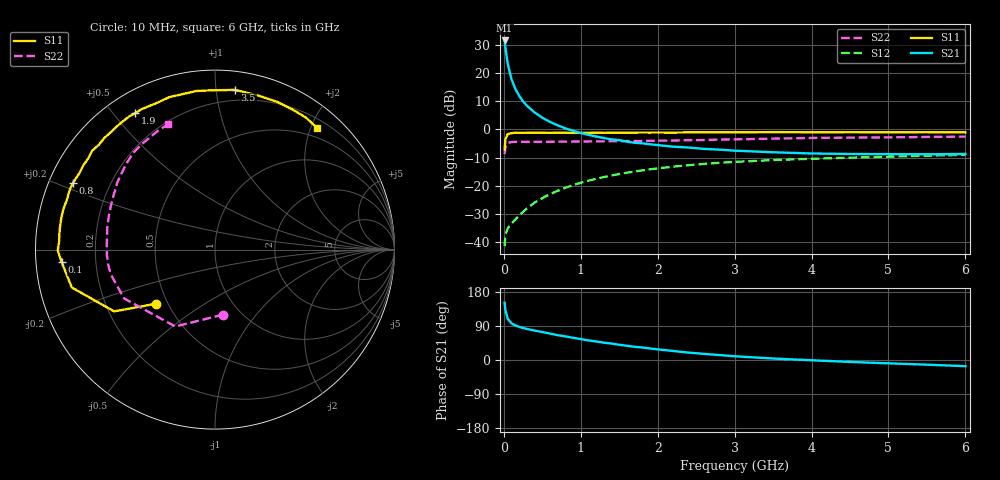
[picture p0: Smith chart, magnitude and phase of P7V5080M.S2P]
! SIEMENS Small Signal Semiconductors
! BFP196
! Si NPN RF Bipolar Junction Transistor in SOT143
! VCE = 0.5 V  IC = 80 mA
! Common Emitter S-Parameters:  May  1996
# GHz  S  MA  R  50
!  f  S11  S21  S12  S22
! GHz  MAG  ANG  MAG  ANG  MAG  ANG  MAG  ANG
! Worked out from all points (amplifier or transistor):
!   36 points, 10 MHz to 6 GHz, reference 50 ohm
!   highest |S21| = 31.7 dB at 10 MHz (marker M1)
!   |S21| within 3 dB of that: start of sweep to 23.11 MHz
!   unconditionally stable (mu >= 1): start of sweep to 13.67 MHz; 160.8 MHz to end of sweep
!   at 250 MHz: K = 1.19, MAG = 17.1 dB, |S12| = -29.4 dB
!   at 1.4 GHz: K = 1.27, MAG = 3.3 dB, |S12| = -16.4 dB
!   at 6 GHz: K = 1.09, MAG = -1.7 dB, |S12| = -9.1 dB
!   S11 on the Smith chart (normalised r, x): 10 MHz: 0.43, -0.33; 100 MHz: 0.08, -0.04; 800 MHz: 0.07, +0.22; 1.9 GHz: 0.08, +0.57; 3.5 GHz: 0.12, +1.12; 6 GHz: 0.33, +2.09
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0.01  0.4441 -137.3  38.64 151.0  0.0083 56.5  0.3649 -82.9
0.02  0.659 -148.5  29.32 131.8  0.0131 44.1  0.4823 -117.3
0.05  0.8254 -165.2  14.99 108.7  0.0173 35.7  0.575 -151.8
0.1  0.8572 -175.4  7.805 96.7  0.0211 41.6  0.5967 -166.6
0.15  0.8761 -179.6  5.272 91.2  0.0248 46.9  0.601 -171.9
0.2  0.8697 177.1  3.967 87.3  0.0293 52.7  0.6013 -174.9
0.25  0.8713 174.5  3.167 84.4  0.034 56.1  0.6032 -177.1
0.3  0.8727 172.5  2.649 82.1  0.039 58.8  0.6023 -178.5
0.4  0.8743 168.2  2.006 77.6  0.0497 61.6  0.6032 179.2
0.5  0.8744 165.1  1.622 73.8  0.0597 62.8  0.6041 177.3
0.6  0.8707 161.2  1.362 69.7  0.0705 63.1  0.604 175.7
0.7  0.8752 157.6  1.184 65.5  0.0806 62.5  0.6051 174.2
0.8  0.8744 154.7  1.045 62.2  0.0912 61.7  0.6064 172.9
1.1  0.8701 144.3  0.802 51.8  0.1221 58.0  0.6123 168.7
1.4  0.8761 134.8  0.664 43.4  0.1509 53.1  0.6165 164.8
1.9  0.8809 120.4  0.545 30.4  0.1944 44.4  0.6275 158.2
2.2  0.879 112.0  0.494 23.9  0.2171 39.2  0.6351 154.1
2.8  0.8897 96.8  0.437 13.0  0.2543 29.0  0.6602 145.7
3.5  0.8967 82.9  0.392 3.9  0.2845 18.1  0.6866 136.4
4.5  0.8932 67.2  0.365 -5.1  0.3145 5.5  0.7155 124.8
5.5  0.8932 55.5  0.361 -12.3  0.3404 -5.1  0.7354 115.3
6  0.8852 50.2  0.366 -16.3  0.352 -10.9  0.7454 110.5
